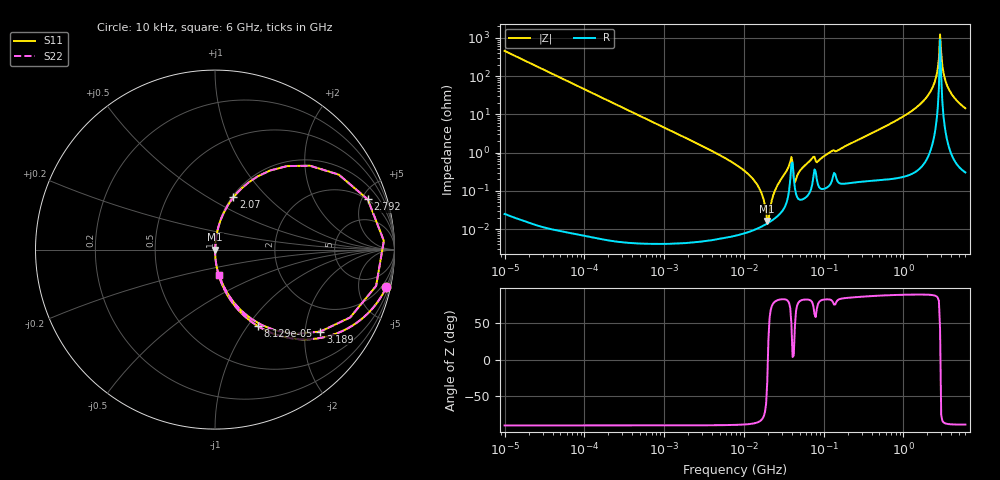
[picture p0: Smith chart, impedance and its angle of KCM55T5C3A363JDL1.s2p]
!Murata Part Number: KCM55T5C3A363JDL1
!These Parameters are Measured in Series Mode Connection
!Data Generated on Mar 13, 2026
!  o--ll--o
!Port1  Port2
!  o------o
!Operation Temp=25[degC], DC Bias Voltage=0[V]
!Freq. Start=10[kHz] Stop=6[GHz] 401[Steps]
# Hz S RI R 50
!Freq.(Hz) S11(Real) S11(Imag) S21(Real) S21(Imag) S12(Real) S12(Imag) S22(Real) S22(Imag)
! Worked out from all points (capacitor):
!   401 points, 10 kHz to 6 GHz, reference 50 ohm
!   read as one part in series: C = 34.9 nF near 10.69 kHz
!   lowest |Z| = 16.3 mohm at 19.66 MHz (marker M1)
!   series resonance near 20.01 MHz, so ESL is about 1.8 nH
!   S11 on the Smith chart (normalised r, x): 10 kHz: 1.00, -9.12; 81.29 kHz: 1.00, -1.12; 2.07 GHz: 1.02, +0.66; 2.792 GHz: 1.96, +5.57; 3.189 GHz: 1.18, -2.41; 6 GHz: 1.01, -0.29
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10000  0.9541 -0.2091  0.0459 0.2091  0.0459 0.2091  0.9541 -0.2091
36591  0.6086 -0.488  0.3914 0.488  0.3914 0.488  0.6086 -0.488
81294  0.2396 -0.4267  0.7604 0.4267  0.7604 0.4267  0.2396 -0.4267
92862  0.1945 -0.3957  0.8055 0.3957  0.8055 0.3957  0.1945 -0.3957
862344  0.00282 -0.0527  0.9972 0.0527  0.9972 0.0527  0.00282 -0.0527
7745967  9.17e-05 -0.00502  0.9999 0.00502  0.9999 0.00502  9.17e-05 -0.00502
1.457263e7  0.000104 -0.00149  0.9999 0.00149  0.9999 0.00149  0.000104 -0.00149
1.965831e7  0.00014 -8.26e-05  0.9999 8.26e-05  0.9999 8.26e-05  0.00014 -8.26e-05
2.101053e7  0.000153 0.000231  0.9998 -0.000231  0.9998 -0.000231  0.000153 0.000231
2.565129e7  0.000208 0.00123  0.9998 -0.00123  0.9998 -0.00123  0.000208 0.00123
3.823436e7  0.00204 0.00547  0.998 -0.00547  0.998 -0.00547  0.00204 0.00547
4.515238e7  0.000824 0.00189  0.9992 -0.00189  0.9992 -0.00189  0.000824 0.00189
7.193098e7  0.0015 0.00693  0.9985 -0.00693  0.9985 -0.00693  0.0015 0.00693
8.494598e7  0.00149 0.0057  0.9985 -0.0057  0.9985 -0.0057  0.00149 0.0057
6.67969e8  0.00501 0.0547  0.995 -0.0547  0.995 -0.0547  0.00501 0.0547
2.069661e9  0.1031 0.2916  0.8969 -0.2916  0.8969 -0.2916  0.1031 0.2916
2.526803e9  0.401 0.4652  0.599 -0.4652  0.599 -0.4652  0.401 0.4652
2.791949e9  0.851 0.2799  0.149 -0.2799  0.149 -0.2799  0.851 0.2799
2.983997e9  0.8978 -0.2019  0.1022 0.2019  0.1022 0.2019  0.8978 -0.2019
3.189254e9  0.5865 -0.4567  0.4135 0.4567  0.4135 0.4567  0.5865 -0.4567
3.89369e9  0.1336 -0.3267  0.8664 0.3267  0.8664 0.3267  0.1336 -0.3267
6e9  0.023 -0.1399  0.977 0.1399  0.977 0.1399  0.023 -0.1399
